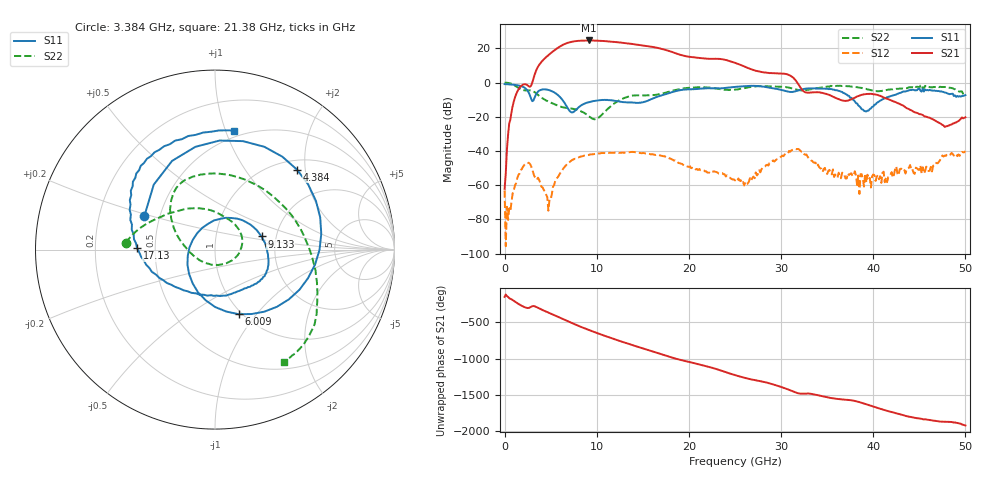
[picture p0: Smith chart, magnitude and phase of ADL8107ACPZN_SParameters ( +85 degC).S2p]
! Analog Devices, Inc.
! Device:	ADL8107ACPZN
! Description:	"GaAs, pHEMT, MMIC, Low Phase Noise Amplifier, 6 GHz to 18 GHz"
! Conditions:	Vdd = 5.0 V
!		IDQ = 90 mA quiescent (Self-biased mode)
!		Pin = -20 dBm
!		Operating Temperature = +85 C (at package bottom)
! Product validation unit SN7 soldered down to Evaluation Board as shown on ADL8107-EVALZ User Guide. Board loss de-embedded from S21 magnitude.  All other RF measurements reference to RF coaxial connector.
! Frequency (GHz)	S11_Mag (dB)	S11_Phase (deg)	S21_Mag (dB)	S21_Phase (deg)	S12_Mag (dB)	S12_Phase (deg)	S22_Mag (dB)	S22_Phase (deg)
#  GHZ  S  DB  R 50
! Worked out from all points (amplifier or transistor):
!   401 points, 10 MHz to 50 GHz, reference 50 ohm
!   highest |S21| = 24.7 dB at 9.133 GHz (marker M1)
!   |S21| within 3 dB of that: 6.186 GHz to 15.11 GHz (8.921 GHz wide, 83.8 % of centre)
!   unconditionally stable (mu >= 1): 36.76 MHz to end of sweep
!   at 8.258 GHz: K = 4.07, MAG = 24.9 dB, |S12| = -43.2 dB
!   at 25.01 GHz: K = 24.76, MAG = 17.4 dB, |S12| = -57.1 dB
!   at 50 GHz: K = 344.38, MAG = -18.4 dB, |S12| = -40.1 dB
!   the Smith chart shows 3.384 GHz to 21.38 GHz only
!   S11 on the Smith chart (normalised r, x): 3.384 GHz: 0.41, +0.19; 4.384 GHz: 1.20, +1.81; 6.009 GHz: 0.97, -0.81; 9.133 GHz: 1.67, +0.26; 17.13 GHz: 0.39, +0.01; 21.38 GHz: 0.44, +1.07
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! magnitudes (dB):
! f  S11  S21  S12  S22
! 10 MHz  -0.8  -62.1  -63.1  0.0
! 384.9 MHz  -0.9  -30.6  -80.3  -0.2
! 1.135 GHz  -1.3  -8.6  -60.1  -1.7
! 2.385 GHz  -3.9  -1.1  -47.1  -4.6
! 3.384 GHz  -7.2  6.4  -55.5  -6.0
! 4.384 GHz  -3.9  14.3  -63.8  -10.0
! 4.884 GHz  -4.5  16.7  -68.4  -11.3
! 6.009 GHz  -8.3  21.1  -53.1  -13.9
! 7.259 GHz  -17.4  23.9  -45.6  -15.2
! 8.383 GHz  -13.0  24.6  -43.1  -17.0
! 9.133 GHz  -11.4  24.7  -42.3  -19.6
! 16.76 GHz  -8.0  20.2  -42.3  -6.8
! 17.13 GHz  -7.2  19.7  -42.8  -6.3
! 21.38 GHz  -3.5  14.3  -51.3  -2.7
! 25.01 GHz  -2.5  11.6  -57.1  -4.1
! 26.25 GHz  -2.0  9.0  -59.2  -3.0
! 31.38 GHz  -5.3  2.6  -39.0  -3.6
! 33.38 GHz  -3.3  -5.7  -45.7  -3.8
! 39.25 GHz  -16.9  -6.6  -58.5  -3.6
! 41.75 GHz  -8.1  -10.0  -55.0  -4.1
! 47.75 GHz  -5.7  -25.9  -42.7  -2.6
! 50 GHz  -7.3  -20.3  -40.1  -7.2
